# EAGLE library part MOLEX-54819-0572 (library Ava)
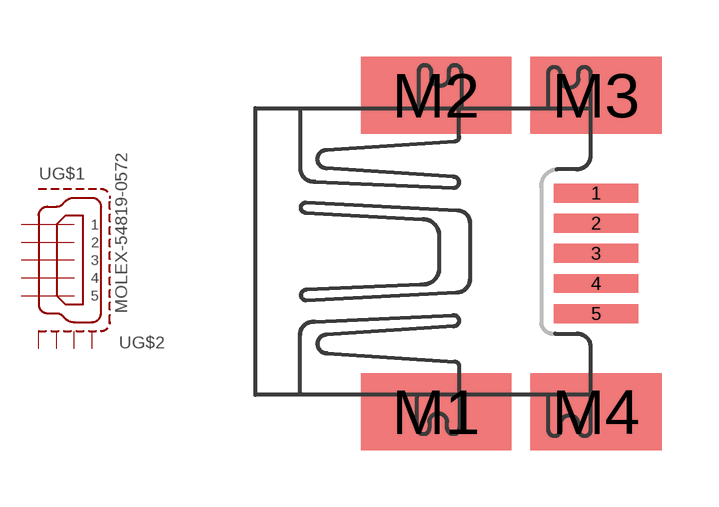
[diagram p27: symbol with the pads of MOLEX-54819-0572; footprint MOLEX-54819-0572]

Designator prefix -; gates G$1=MOLEX-54819-0572 G$2=MINIUSBSHEILD

## MOLEX-54819-0572  [MOLEX-54819-0572]
1  G$1:1  in
2  G$1:2  in
3  G$1:3  in
4  G$1:4  in
5  G$1:5  in
M1  G$2:S1  pas
M2  G$2:S2  pas
M3  G$2:S3  pas
M4  G$2:S4  pas

## Footprint MOLEX-54819-0572 (pad centres in mm)
smd 2.25 x 0.5: 1 0,1.6; 2 0,0.8; 3 0,0; 4 0,-0.8; 5 0,-1.6
smd 4 x 2.05: M1 -4.25,-4.2; M2 -4.25,4.2
smd 3.5 x 2.05: M3 0,4.2; M4 0,-4.2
